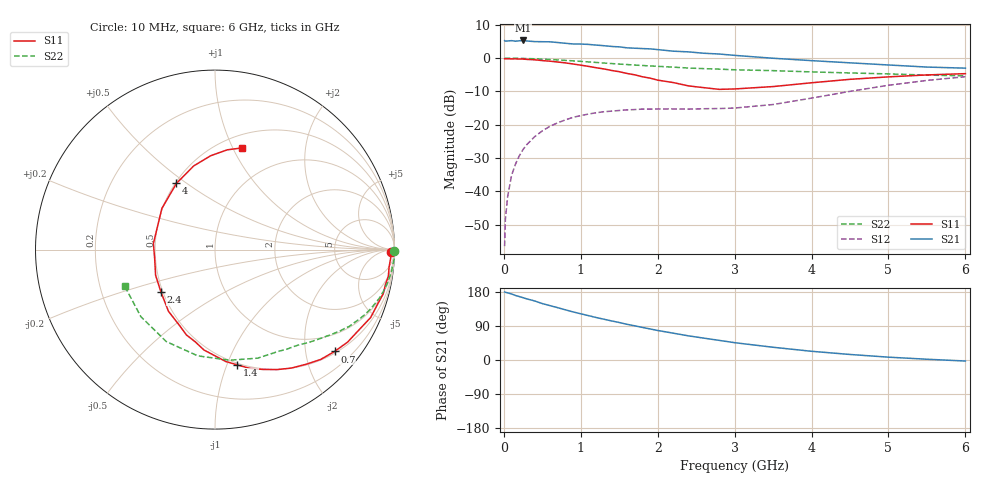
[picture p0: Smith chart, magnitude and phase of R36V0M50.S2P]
! SIEMENS Small Signal Semiconductors
! BFR181
! Si NPN RF Bipolar Junction Transistor in SOT23
! VCE = 6 V  IC = 0.5 mA
! Common Emitter S-Parameters:  May  1996
# GHz  S  MA  R  50
!  f  S11  S21  S12  S22
! GHz  MAG  ANG  MAG  ANG  MAG  ANG  MAG  ANG
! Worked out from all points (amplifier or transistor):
!   36 points, 10 MHz to 6 GHz, reference 50 ohm
!   highest |S21| = 5.3 dB at 250 MHz (marker M1)
!   |S21| within 3 dB of that: start of sweep to 2.108 GHz
!   unconditionally stable (mu >= 1): 2.38 GHz to 3.951 GHz
!   at 250 MHz: K = 0.11, MSG = 16.4 dB, |S12| = -27.4 dB
!   at 1.4 GHz: K = 0.60, MSG = 9.7 dB, |S12| = -15.9 dB
!   at 6 GHz: K = 0.91, MSG = 1.3 dB, |S12| = -5.6 dB
!   S11 on the Smith chart (normalised r, x): 10 MHz: 65, -40; 700 MHz: 0.54, -2.62; 1.4 GHz: 0.48, -1.09; 2.4 GHz: 0.49, -0.27; 4 GHz: 0.51, +0.46; 6 GHz: 0.63, +1.08
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0.01  0.978 -0.8  1.833 179.6  0.0015 95.2  0.9999 -0.3
0.02  0.9782 -1.2  1.801 178.7  0.0038 84.2  0.9989 -0.6
0.05  0.9799 -2.8  1.811 177.1  0.0084 89.7  0.9983 -1.4
0.1  0.9748 -5.7  1.834 174.3  0.0173 85.9  0.9999 -2.8
0.15  0.9773 -8.8  1.799 170.3  0.0254 83.6  0.9959 -4.3
0.25  0.9693 -14.7  1.845 164.4  0.0425 79.8  0.9914 -7.0
0.4  0.946 -23.6  1.773 155.9  0.066 73.8  0.979 -11.0
0.5  0.9192 -29.0  1.767 148.9  0.0809 70.0  0.9676 -13.7
0.7  0.8754 -40.4  1.718 138.1  0.1071 62.4  0.9399 -18.8
0.9  0.8173 -51.3  1.634 126.9  0.1292 55.7  0.9114 -23.3
1.1  0.7525 -62.7  1.61 117.1  0.1447 50.0  0.8777 -27.5
1.4  0.654 -79.1  1.5 103.1  0.1601 42.8  0.83 -33.2
1.9  0.5014 -108.5  1.379 82.0  0.1715 36.1  0.7638 -40.7
2.2  0.4306 -127.0  1.274 70.9  0.1725 34.5  0.7332 -45.0
2.4  0.3833 -141.7  1.243 63.7  0.1716 35.1  0.7111 -48.0
3  0.3448 174.4  1.102 45.7  0.1781 40.6  0.6692 -57.7
3.5  0.3745 142.2  0.997 33.6  0.2011 47.1  0.6497 -68.6
4  0.4269 120.2  0.918 23.0  0.2511 51.6  0.6217 -82.5
4.5  0.4811 104.3  0.851 14.6  0.3174 50.5  0.5997 -99.2
5  0.5237 92.6  0.79 7.5  0.3916 45.6  0.5799 -117.9
5.5  0.56 83.0  0.735 2.0  0.4633 38.0  0.5569 -137.9
6  0.5854 75.3  0.708 -2.7  0.5262 29.4  0.5427 -158.0
